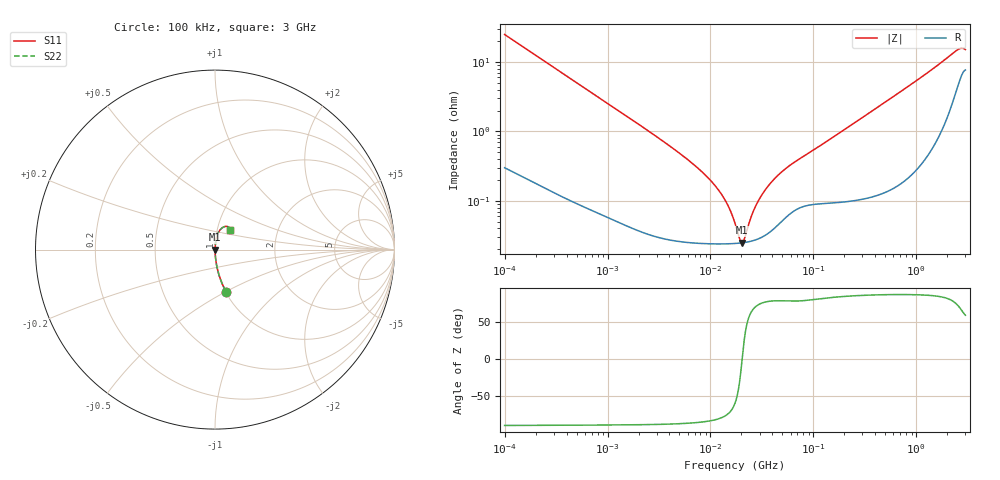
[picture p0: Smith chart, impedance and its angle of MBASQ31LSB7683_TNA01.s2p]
! MBASQ31LSB7683_TNA01  S-PARAMETER MODEL  ( Standard Model )
! Model Generated by TAIYO YUDEN Corporation (http://www.ty-top.com)
! Version 1.0
! TAIYO YUDEN Control No. 220601
! Copyright(c) 2013 TAIYO YUDEN CO.,LTD. All Rights Reserved.
! Product Description (link to TY-COMPAS)
! https://ds.yuden.co.jp/TYCOMPAS/or/detail?pn=MBASQ31LSB7683KTNA01&u=M
! Products Name : Multilayer Ceramic Capacitors
! Characteristics :
!  Capacitance : 0.068 [uF] , Rated Voltage : 250 [V] , TCC : X7R
!  Case Size : 3.2 x 1.6 / 0.126 x 0.063 [mm/inch] , Thickness : 1.6 / 0.063 [mm/inch]
!  (Conditions: Temperature = 25 [degC] , DC Bias Voltage = 0 [V])
! External Node Assignments :
!  1  o---| |---o  2
! GND o---------o GND
! Frequency Range : 100kHz  -  3GHz  [ 401 STEP ]
# MHZ S RI R 50
! Freq[MHz].  S11 Real  S11 Imag  S21 Real  S21 Imag  S12 Real  S12 Imag  S22 Real  S22 Imag
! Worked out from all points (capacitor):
!   401 points, 100 kHz to 3 GHz, reference 50 ohm
!   read as one part in series: C = 63.7 nF near 105.3 kHz
!   lowest |Z| = 24.8 mohm at 20.22 MHz (marker M1)
!   series resonance near 20.31 MHz, so ESL is about 960 pH
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0.1  0.061 -0.2335  0.939 0.2335  0.939 0.2335  0.061 -0.2335
0.222319  0.0142 -0.1111  0.9858 0.1111  0.9858 0.1111  0.0142 -0.1111
0.562235  0.00285 -0.0448  0.9971 0.0448  0.9971 0.0448  0.00285 -0.0448
3.161081  0.000358 -0.00794  0.9996 0.00794  0.9996 0.00794  0.000358 -0.00794
6.674626  0.000259 -0.00345  0.9997 0.00345  0.9997 0.00345  0.000259 -0.00345
10.61445  0.000243 -0.00177  0.9998 0.00177  0.9998 0.00177  0.000243 -0.00177
14.46142  0.00024 -0.000884  0.9998 0.000884  0.9998 0.000884  0.00024 -0.000884
16.0318  0.000241 -0.00061  0.9998 0.00061  0.9998 0.00061  0.000241 -0.00061
17.7727  0.000243 -0.000342  0.9998 0.000342  0.9998 0.000342  0.000243 -0.000342
19.20135  0.000246 -0.000144  0.9998 0.000144  0.9998 0.000144  0.000246 -0.000144
20.21703  0.000248 -1.13e-05  0.9998 1.13e-05  0.9998 1.13e-05  0.000248 -1.13e-05
21.28644  0.00025 0.000121  0.9997 -0.000121  0.9997 -0.000121  0.00025 0.000121
24.84619  0.000262 0.000523  0.9997 -0.000523  0.9997 -0.000523  0.000262 0.000523
27.54426  0.000274 0.000799  0.9997 -0.000799  0.9997 -0.000799  0.000274 0.000799
35.64176  0.000334 0.00153  0.9997 -0.00153  0.9997 -0.00153  0.000334 0.00153
52.46276  0.000559 0.00277  0.9994 -0.00277  0.9994 -0.00277  0.000559 0.00277
97.38194  0.000906 0.00516  0.9991 -0.00516  0.9991 -0.00516  0.000906 0.00516
547.5153  0.00224 0.0289  0.9978 -0.0289  0.9978 -0.0289  0.00224 0.0289
1535  0.0137 0.083  0.9863 -0.083  0.9863 -0.083  0.0137 0.083
2378.954  0.0492 0.1266  0.9508 -0.1266  0.9508 -0.1266  0.0492 0.1266
2706.139  0.0739 0.1271  0.9261 -0.1271  0.9261 -0.1271  0.0739 0.1271
3000  0.0847 0.1105  0.9153 -0.1105  0.9153 -0.1105  0.0847 0.1105
